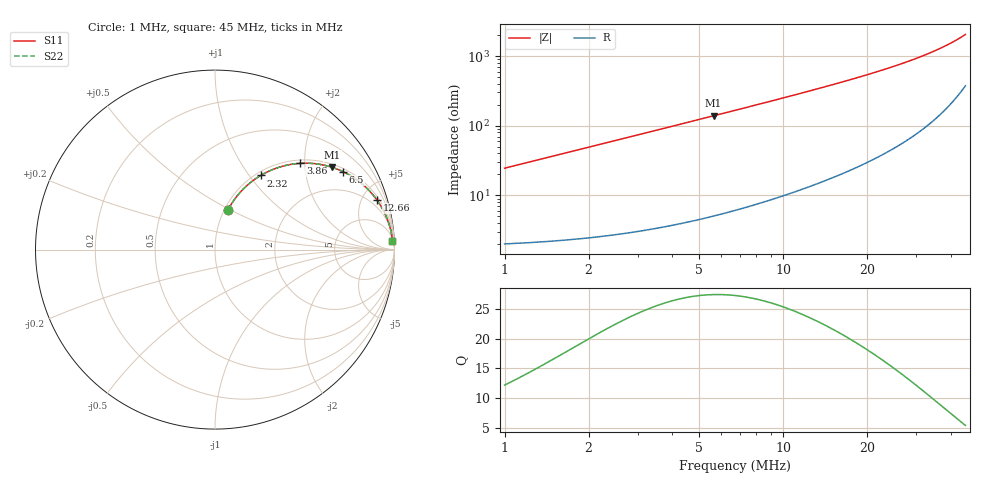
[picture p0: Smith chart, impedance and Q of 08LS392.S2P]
! Coilcraft 0805LS-392 Chip Inductor
! 18 September 2002
# MHZ S MA R 50
!Freq  MagS11  AngS11  MagS21  AngS21  MagS12  AngS12  MagS22  AngS22
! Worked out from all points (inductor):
!   401 points, 1 MHz to 45 MHz, reference 50 ohm
!   read as one part in series: L = 3.9 uH near 1.22 MHz
!   highest Q = 27.4 at 5.62 MHz (marker M1), where L = 3.93 uH
!   S11 on the Smith chart (normalised r, x): 1 MHz: 1.04, +0.49; 2.32 MHz: 1.05, +1.14; 3.86 MHz: 1.07, +1.90; 6.5 MHz: 1.12, +3.22; 12.66 MHz: 1.28, +6.44; 45 MHz: 8, +40
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1  0.2344 71.8  0.9532 -13.5  0.9532 -13.5  0.2344 71.8
1.22  0.2818 69.7  0.94 -16.3  0.94 -16.3  0.2818 69.7
1.44  0.3271 67.4  0.925 -19.1  0.925 -19.1  0.3271 67.4
1.66  0.3703 65.1  0.9084 -21.7  0.9084 -21.7  0.3703 65.1
1.99  0.4306 61.7  0.8812 -25.5  0.8812 -25.5  0.4306 61.7
2.32  0.4855 58.3  0.8521 -29.0  0.8521 -29.0  0.4855 58.3
2.65  0.535 55.2  0.822 -32.3  0.822 -32.3  0.535 55.2
3.09  0.5932 51.3  0.7813 -36.3  0.7813 -36.3  0.5932 51.3
3.86  0.6758 45.3  0.7118 -42.5  0.7118 -42.5  0.6758 45.3
4.74  0.7461 39.7  0.6389 -48.2  0.6389 -48.2  0.7461 39.7
5.62  0.7976 35.1  0.5749 -52.9  0.5749 -52.9  0.7976 35.1
6.5  0.8357 31.3  0.5195 -56.6  0.5195 -56.6  0.8357 31.3
7.38  0.8644 28.1  0.4719 -59.7  0.4719 -59.7  0.8644 28.1
8.37  0.8886 25.2  0.4263 -62.6  0.4263 -62.6  0.8886 25.2
10.24  0.9198 20.9  0.3577 -66.8  0.3577 -66.8  0.9198 20.9
12.66  0.9437 17.0  0.293 -70.5  0.293 -70.5  0.9437 17.0
15.74  0.9609 13.6  0.235 -73.7  0.235 -73.7  0.9609 13.6
19.15  0.9718 10.9  0.1896 -76.0  0.1896 -76.0  0.9718 10.9
23  0.9789 8.8  0.1526 -77.7  0.1526 -77.7  0.9789 8.8
30.37  0.9858 6.0  0.1045 -79.2  0.1045 -79.2  0.9858 6.0
37.74  0.9888 4.1  0.07213 -79.0  0.07213 -79.0  0.9888 4.1
45  0.99 2.7  0.04852 -76.7  0.04852 -76.7  0.99 2.7
